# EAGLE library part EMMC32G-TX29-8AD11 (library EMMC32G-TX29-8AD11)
eMMC 32GB eMMC 5.1 (HS400) 153B Source: Datasheet
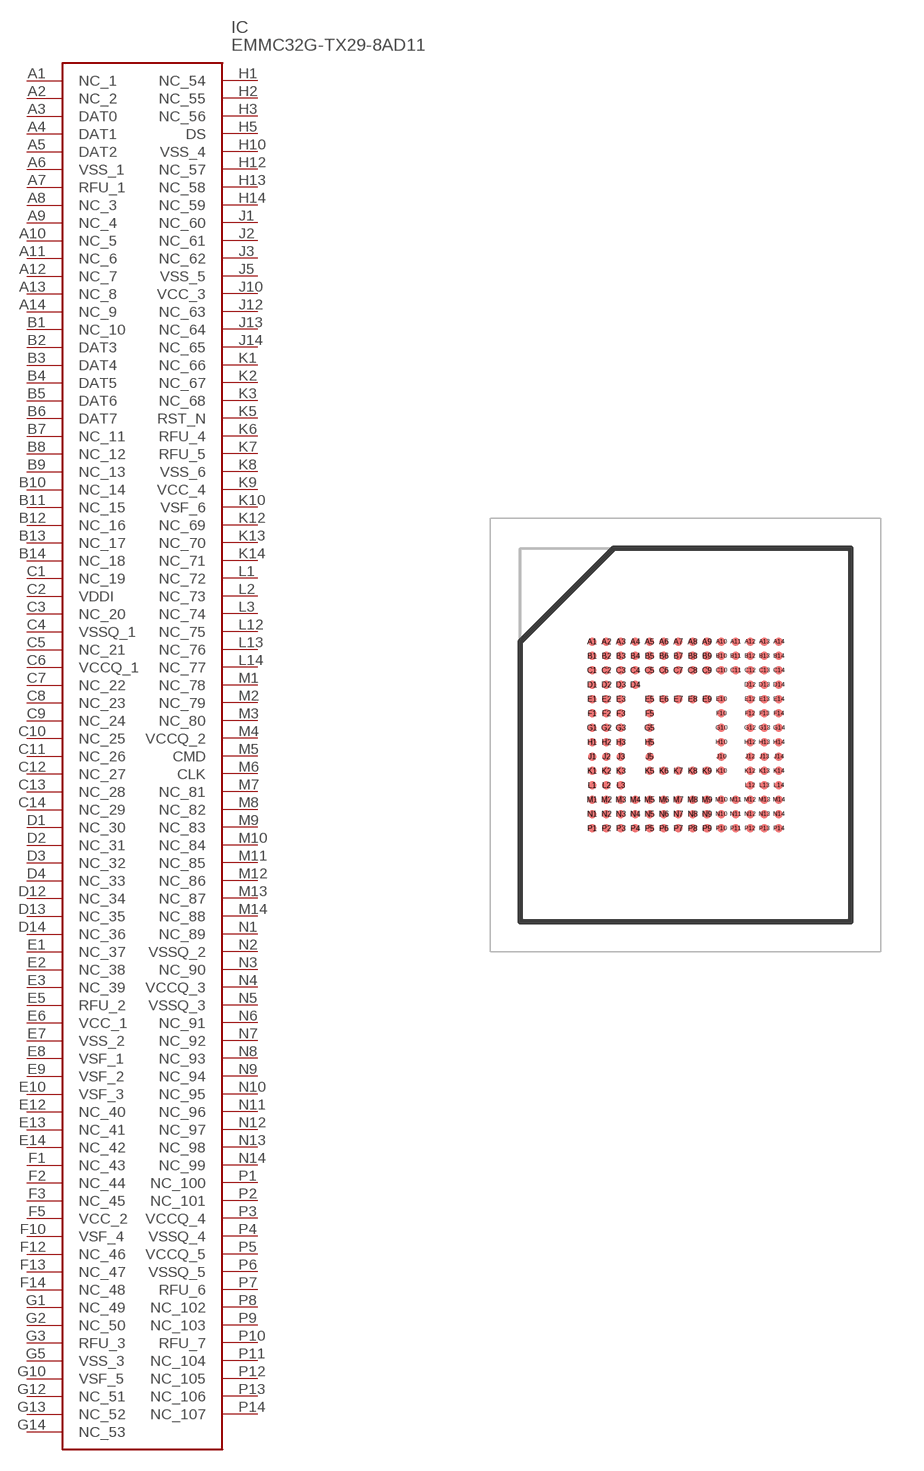
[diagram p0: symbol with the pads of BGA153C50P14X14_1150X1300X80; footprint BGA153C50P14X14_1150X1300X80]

Designator prefix IC

## EMMC32G-TX29-8AD11 (Description: eMMC 32GB eMMC 5.1 (HS400) 153B; Height: 0.8mm; Manufacturer_Name: Kingston Technology; Manufacturer_Part_Number: EMMC32G-TX29-8AD11; Mouser_Part_Number: 524-TX29-8AD11; Mouser_Price-Stock: https://www.mouser.co.uk/ProductDetail/Kingston/EMMC32G-TX29-8AD11?qs=4ASt3YYao0WliodWhJOwmQ%3D%3D)  [BGA153C50P14X14_1150X1300X80]
A1  NC_1
A2  NC_2
A3  DAT0
A4  DAT1
A5  DAT2
A6  VSS_1
A7  RFU_1
A8  NC_3
A9  NC_4
A10  NC_5
A11  NC_6
A12  NC_7
A13  NC_8
A14  NC_9
B1  NC_10
B2  DAT3
B3  DAT4
B4  DAT5
B5  DAT6
B6  DAT7
B7  NC_11
B8  NC_12
B9  NC_13
B10  NC_14
B11  NC_15
B12  NC_16
B13  NC_17
B14  NC_18
C1  NC_19
C2  VDDI
C3  NC_20
C4  VSSQ_1
C5  NC_21
C6  VCCQ_1
C7  NC_22
C8  NC_23
C9  NC_24
C10  NC_25
C11  NC_26
C12  NC_27
C13  NC_28
C14  NC_29
D1  NC_30
D2  NC_31
D3  NC_32
D4  NC_33
D12  NC_34
D13  NC_35
D14  NC_36
E1  NC_37
E2  NC_38
E3  NC_39
E5  RFU_2
E6  VCC_1
E7  VSS_2
E8  VSF_1
E9  VSF_2
E10  VSF_3
E12  NC_40
E13  NC_41
E14  NC_42
F1  NC_43
F2  NC_44
F3  NC_45
F5  VCC_2
F10  VSF_4
F12  NC_46
F13  NC_47
F14  NC_48
G1  NC_49
G2  NC_50
G3  RFU_3
G5  VSS_3
G10  VSF_5
G12  NC_51
G13  NC_52
G14  NC_53
H1  NC_54
H2  NC_55
H3  NC_56
H5  DS
H10  VSS_4
H12  NC_57
H13  NC_58
H14  NC_59
J1  NC_60
J2  NC_61
J3  NC_62
J5  VSS_5
J10  VCC_3
J12  NC_63
J13  NC_64
J14  NC_65
K1  NC_66
K2  NC_67
K3  NC_68
K5  RST_N
K6  RFU_4
K7  RFU_5
K8  VSS_6
K9  VCC_4
K10  VSF_6
K12  NC_69
K13  NC_70
K14  NC_71
L1  NC_72
L2  NC_73
L3  NC_74
L12  NC_75
L13  NC_76
L14  NC_77
M1  NC_78
M2  NC_79
M3  NC_80
M4  VCCQ_2
M5  CMD
M6  CLK
M7  NC_81
M8  NC_82
M9  NC_83
M10  NC_84
M11  NC_85
M12  NC_86
M13  NC_87
M14  NC_88
N1  NC_89
N2  VSSQ_2
N3  NC_90
N4  VCCQ_3
N5  VSSQ_3
N6  NC_91
N7  NC_92
N8  NC_93
N9  NC_94
N10  NC_95
N11  NC_96
N12  NC_97
N13  NC_98
N14  NC_99
P1  NC_100
P2  NC_101
P3  VCCQ_4
P4  VSSQ_4
P5  VCCQ_5
P6  VSSQ_5
P7  RFU_6
P8  NC_102
P9  NC_103
P10  RFU_7
P11  NC_104
P12  NC_105
P13  NC_106
P14  NC_107

## Footprint BGA153C50P14X14_1150X1300X80 (pad centres in mm)
EMMC32G-TX29-8AD11
smd 0.29 x 0.29: A1 -3.25,3.25; A2 -2.75,3.25; A3 -2.25,3.25; A4 -1.75,3.25; A5 -1.25,3.25; A6 -0.75,3.25; A7 -0.25,3.25; A8 0.25,3.25; A9 0.75,3.25; A10 1.25,3.25; A11 1.75,3.25; A12 2.25,3.25; A13 2.75,3.25; A14 3.25,3.25; B1 -3.25,2.75; B2 -2.75,2.75; B3 -2.25,2.75; B4 -1.75,2.75; B5 -1.25,2.75; B6 -0.75,2.75; B7 -0.25,2.75; B8 0.25,2.75; B9 0.75,2.75; B10 1.25,2.75; B11 1.75,2.75; B12 2.25,2.75; B13 2.75,2.75; B14 3.25,2.75; C1 -3.25,2.25; C2 -2.75,2.25; C3 -2.25,2.25; C4 -1.75,2.25; C5 -1.25,2.25; C6 -0.75,2.25; C7 -0.25,2.25; C8 0.25,2.25; C9 0.75,2.25; C10 1.25,2.25; C11 1.75,2.25; C12 2.25,2.25; C13 2.75,2.25; C14 3.25,2.25; D1 -3.25,1.75; D2 -2.75,1.75; D3 -2.25,1.75; D4 -1.75,1.75; D12 2.25,1.75; D13 2.75,1.75; D14 3.25,1.75; E1 -3.25,1.25; E2 -2.75,1.25; E3 -2.25,1.25; E5 -1.25,1.25; E6 -0.75,1.25; E7 -0.25,1.25; E8 0.25,1.25; E9 0.75,1.25; E10 1.25,1.25; E12 2.25,1.25; E13 2.75,1.25; E14 3.25,1.25; F1 -3.25,0.75; F2 -2.75,0.75; F3 -2.25,0.75; F5 -1.25,0.75; F10 1.25,0.75; F12 2.25,0.75; F13 2.75,0.75; F14 3.25,0.75; G1 -3.25,0.25; G2 -2.75,0.25; G3 -2.25,0.25; G5 -1.25,0.25; G10 1.25,0.25; G12 2.25,0.25; G13 2.75,0.25; G14 3.25,0.25; H1 -3.25,-0.25; H2 -2.75,-0.25; H3 -2.25,-0.25; H5 -1.25,-0.25; H10 1.25,-0.25; H12 2.25,-0.25; H13 2.75,-0.25; H14 3.25,-0.25; J1 -3.25,-0.75; J2 -2.75,-0.75; J3 -2.25,-0.75; J5 -1.25,-0.75; J10 1.25,-0.75; J12 2.25,-0.75; J13 2.75,-0.75; J14 3.25,-0.75; K1 -3.25,-1.25; K2 -2.75,-1.25; K3 -2.25,-1.25; K5 -1.25,-1.25; K6 -0.75,-1.25; K7 -0.25,-1.25; K8 0.25,-1.25; K9 0.75,-1.25; K10 1.25,-1.25; K12 2.25,-1.25; K13 2.75,-1.25; K14 3.25,-1.25; L1 -3.25,-1.75; L2 -2.75,-1.75; L3 -2.25,-1.75; L12 2.25,-1.75; L13 2.75,-1.75; L14 3.25,-1.75; M1 -3.25,-2.25; M2 -2.75,-2.25; M3 -2.25,-2.25; M4 -1.75,-2.25; M5 -1.25,-2.25; M6 -0.75,-2.25; M7 -0.25,-2.25; M8 0.25,-2.25; M9 0.75,-2.25; M10 1.25,-2.25; M11 1.75,-2.25; M12 2.25,-2.25; M13 2.75,-2.25; M14 3.25,-2.25; N1 -3.25,-2.75; N2 -2.75,-2.75; N3 -2.25,-2.75; N4 -1.75,-2.75; N5 -1.25,-2.75; N6 -0.75,-2.75; N7 -0.25,-2.75; N8 0.25,-2.75; N9 0.75,-2.75; N10 1.25,-2.75; N11 1.75,-2.75; N12 2.25,-2.75; N13 2.75,-2.75; N14 3.25,-2.75; P1 -3.25,-3.25; P2 -2.75,-3.25; P3 -2.25,-3.25; P4 -1.75,-3.25; P5 -1.25,-3.25; P6 -0.75,-3.25; P7 -0.25,-3.25; P8 0.25,-3.25; P9 0.75,-3.25; P10 1.25,-3.25; P11 1.75,-3.25; P12 2.25,-3.25; P13 2.75,-3.25; P14 3.25,-3.25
